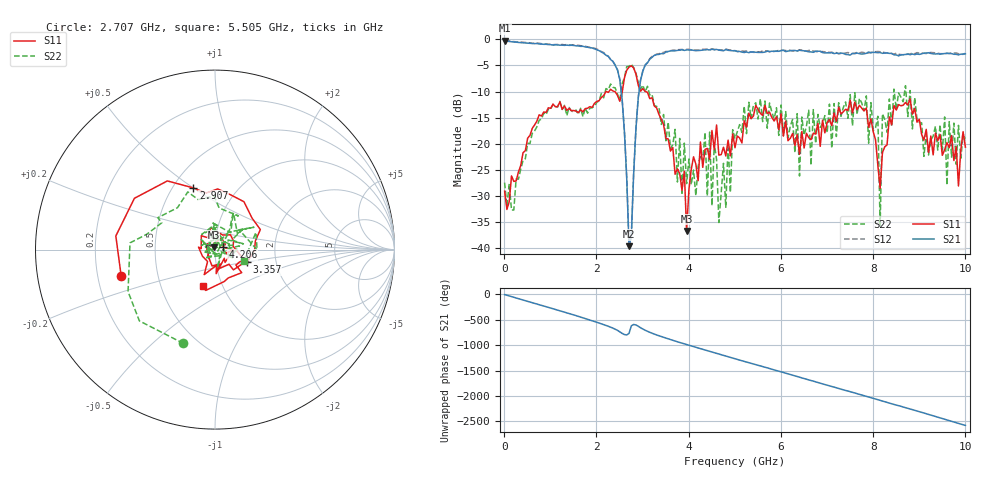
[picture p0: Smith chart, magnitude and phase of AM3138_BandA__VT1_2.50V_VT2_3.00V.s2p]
! Date/Time: Tue, Nov 13, 2018 4:42 PM
! Network Analyzer: Agilent Technologies E8364B Rev: A.07.50.67
! Sweep from 0.010 to 10.000 GHz, 201 Points, Sweep Type: LIN
! Power Supply: 2.501 V, 0.000 A
# Hz S DB R 50
!freq MagS11 AngS11 MagS21 AngS21 MagS12 AngS12 MagS22 AngS22
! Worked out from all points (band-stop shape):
!   201 points, 10 MHz to 10 GHz, reference 50 ohm
!   highest |S21| = -0.25 dB at 10 MHz (marker M1); lowest = -39.6 dB at 2.707 GHz (marker M2)
!   |S21| within 3 dB of the highest: start of sweep to 2.258 GHz; 3.232 GHz to end of sweep
!   lowest |S11| = -36.7 dB at 3.956 GHz (marker M3), VSWR 1.03, Z = 49.2 + j1.19 ohm
!   |S11| at or under -10 dB: start of sweep to 2.205 GHz; 2.398 GHz to 2.562 GHz (164.1 MHz wide, 6.62 % of centre); 3.068 GHz to end of sweep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
!   |S22| runs from -35.7 to -4.7 dB; largest |S21 - S12| = 0.034
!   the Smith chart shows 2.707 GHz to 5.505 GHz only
!   S11 on the Smith chart (normalised r, x): 2.707 GHz: 0.30, -0.13; 2.907 GHz: 0.63, +0.50; 3.357 GHz: 1.41, -0.21; 4.206 GHz: 1.09, +0.03; 5.505 GHz: 0.81, -0.35
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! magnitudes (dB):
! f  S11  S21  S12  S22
! 10 MHz  -29.0  -0.3  -0.2  -27.4
! 1.708 GHz  -13.9  -1.3  -1.3  -14.8
! 2.508 GHz  -11.8  -7.7  -7.6  -11.7
! 2.707 GHz  -5.3  -39.6  -39.3  -5.2
! 2.907 GHz  -8.8  -11.2  -11.1  -8.2
! 3.357 GHz  -14.4  -2.9  -2.8  -13.1
! 3.956 GHz  -36.7  -2.0  -1.9  -27.6
! 4.206 GHz  -27.1  -2.1  -2.1  -24.3
! 4.506 GHz  -17.4  -1.9  -1.8  -31.8
! 4.555 GHz  -21.2  -2.0  -1.9  -19.9
! 4.655 GHz  -22.1  -2.1  -2.0  -35.0
! 5.005 GHz  -20.8  -2.1  -2.2  -19.0
! 5.505 GHz  -13.4  -2.5  -2.4  -15.2
! 6.354 GHz  -18.2  -2.2  -2.2  -14.2
! 6.404 GHz  -22.0  -2.1  -2.0  -26.1
! 6.703 GHz  -17.9  -2.5  -2.2  -13.4
! 7.952 GHz  -15.2  -2.6  -2.5  -12.1
! 8.102 GHz  -24.1  -2.6  -2.3  -14.7
! 8.152 GHz  -28.5  -2.5  -2.4  -35.7
! 8.202 GHz  -21.6  -2.7  -2.5  -14.2
! 8.352 GHz  -14.8  -2.7  -2.7  -11.4
! 10 GHz  -20.6  -2.8  -2.7  -19.0
